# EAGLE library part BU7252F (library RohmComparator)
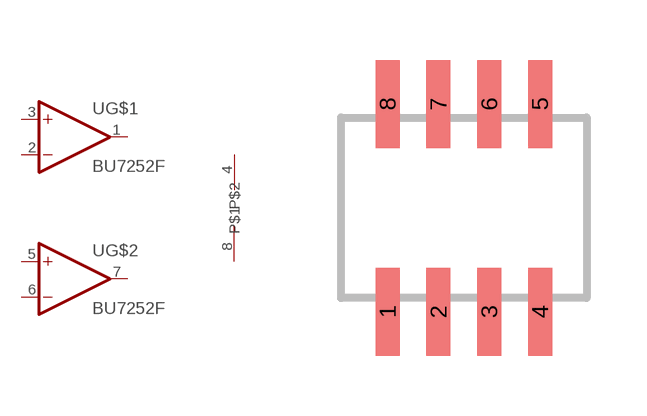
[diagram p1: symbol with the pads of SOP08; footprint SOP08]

Designator prefix -; gates G$1=OPAMP G$2=OPAMP G$3=SUPPLY

## BU7252F  [SOP08]
1  G$1:OUT  out
2  G$1:-IN  in
3  G$1:+IN  in
4  G$3:P$1
5  G$2:+IN  in
6  G$2:-IN  in
7  G$2:OUT  out
8  G$3:P$2

## Footprint SOP08 (pad centres in mm)
smd 0.6 x 2.2: 1 -1.905,-2.6; 2 -0.635,-2.6; 3 0.635,-2.6; 4 1.905,-2.6; 5 1.905,2.6; 6 0.635,2.6; 7 -0.635,2.6; 8 -1.905,2.6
